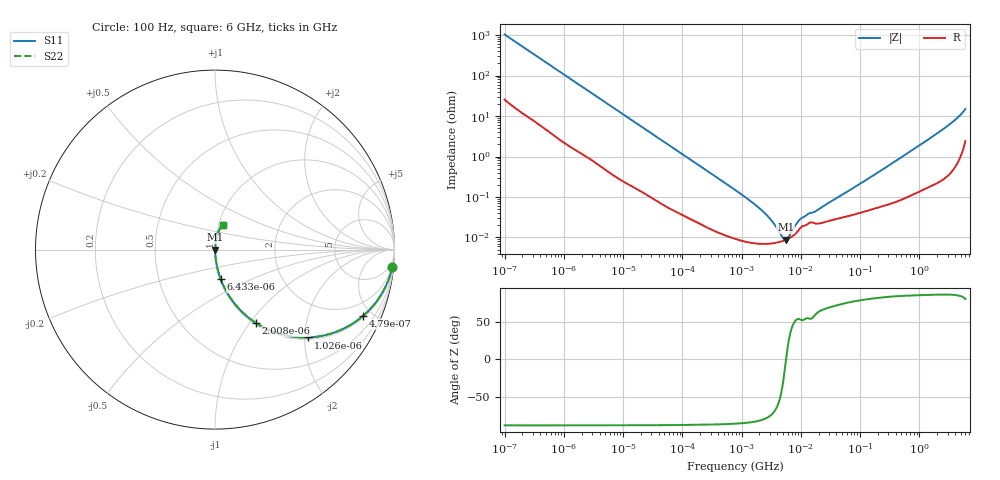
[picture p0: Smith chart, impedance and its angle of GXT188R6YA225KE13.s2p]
!Murata Part Number: GXT188R6YA225KE13
!These Parameters are Measured in Series Mode Connection
!Data Generated on Jan 08, 2026
!  o--ll--o
!Port1  Port2
!  o------o
!Operation Temp=25[degC], DC Bias Voltage=0[V]
!Freq. Start=100[Hz] Stop=6[GHz] 401[Steps]
# Hz S RI R 50
!Freq.(Hz) S11(Real) S11(Imag) S21(Real) S21(Imag) S12(Real) S12(Imag) S22(Real) S22(Imag)
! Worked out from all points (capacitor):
!   401 points, 100 Hz to 6 GHz, reference 50 ohm
!   read as one part in series: C = 1.53 uF near 109 Hz
!   lowest |Z| = 8.74 mohm at 5.555 MHz (marker M1)
!   series resonance near 5.641 MHz, so ESL is about 520 pH
!   S11 on the Smith chart (normalised r, x): 100 Hz: 2, -21; 479 Hz: 1.10, -4.41; 1.026 kHz: 1.04, -2.08; 2.008 kHz: 1.02, -1.07; 6.433 kHz: 1.01, -0.34; 6 GHz: 1.05, +0.29
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100  0.9885 -0.0951  0.0115 0.0951  0.0115 0.0951  0.9885 -0.0951
245  0.9438 -0.2193  0.0562 0.2193  0.0562 0.2193  0.9438 -0.2193
479  0.8244 -0.3697  0.1756 0.3697  0.1756 0.3697  0.8244 -0.3697
750  0.665 -0.4617  0.335 0.4617  0.335 0.4617  0.665 -0.4617
1026  0.5197 -0.4894  0.4803 0.4894  0.4803 0.4894  0.5197 -0.4894
2008  0.2283 -0.409  0.7717 0.409  0.7717 0.409  0.2283 -0.409
3437  0.0959 -0.2836  0.9041 0.2836  0.9041 0.2836  0.0959 -0.2836
6433  0.0315 -0.1642  0.9685 0.1642  0.9685 0.1642  0.0315 -0.1642
14402  0.00762 -0.076  0.9924 0.076  0.9924 0.076  0.00762 -0.076
40335  0.00151 -0.0278  0.9985 0.0278  0.9985 0.0278  0.00151 -0.0278
774597  9.48e-05 -0.0015  0.9999 0.0015  0.9999 0.0015  9.48e-05 -0.0015
2268635  6.94e-05 -0.000442  0.9999 0.000442  0.9999 0.000442  6.94e-05 -0.000442
3245845  7.12e-05 -0.000246  0.9999 0.000246  0.9999 0.000246  7.12e-05 -0.000246
4643984  7.94e-05 -8.27e-05  0.9999 8.27e-05  0.9999 8.27e-05  7.94e-05 -8.27e-05
5554849  8.72e-05 -6.4e-06  0.9999 6.4e-06  0.9999 6.4e-06  8.72e-05 -6.4e-06
6353432  9.58e-05 5.04e-05  0.9999 -5.04e-05  0.9999 -5.04e-05  9.58e-05 5.04e-05
9506416  0.000162 0.00022  0.9998 -0.00022  0.9998 -0.00022  0.000162 0.00022
1.555665e7  0.000235 0.000336  0.9998 -0.000336  0.9998 -0.000336  0.000235 0.000336
3.124326e8  0.0007 0.00609  0.9993 -0.00609  0.9993 -0.00609  0.0007 0.00609
2.450438e9  0.00471 0.0456  0.9953 -0.0456  0.9953 -0.0456  0.00471 0.0456
4.009986e9  0.0117 0.0787  0.9883 -0.0787  0.9883 -0.0787  0.0117 0.0787
6e9  0.0433 0.1377  0.9567 -0.1377  0.9567 -0.1377  0.0433 0.1377
